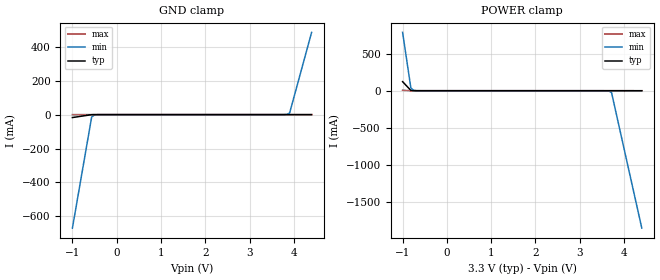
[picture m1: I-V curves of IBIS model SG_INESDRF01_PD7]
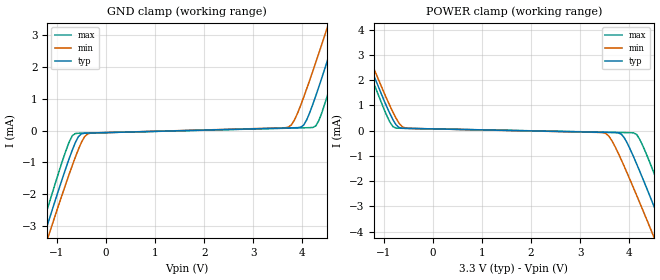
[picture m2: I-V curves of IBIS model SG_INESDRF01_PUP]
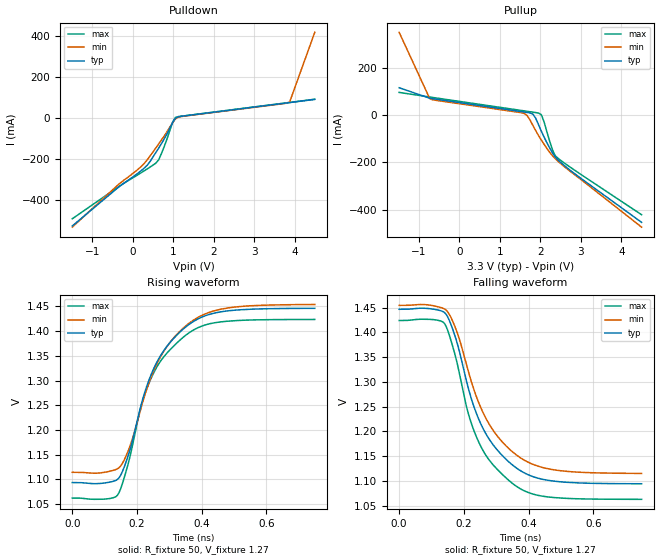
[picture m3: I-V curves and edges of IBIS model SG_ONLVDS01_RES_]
|   This file is an IBIS representation of the   |
|   Integrated Device Technology , Inc.   |
|   ICS854S058i   |
|   8:1 DIFFERENTIAL-TO-LVDS CLOCK MULTIPLIER   |
[IBIS Ver]   4.1
[File name]   854s058i_3v3.ibs
[File Rev]   1.0
[Date]   15 Jan 2010
[Source]   Originated at Integrated Device Technology, Inc.
[Disclaimer]
IDT hereby grants the user of this IBIS model a non-exclusive,
nontransferable license to use this IBIS model under the following terms.
Before using this IBIS model, the user should read this license.
If the user does not accept these terms,  the IBIS model should be
returned to IDT within 30 days.
   The user is granted this license only to use the IBIS model and
is not granted rights to sell, load, rent, lease or license the IBIS
model in whole or in part, or in modified form to anyone other than
user. User may modify the IBIS model to suit its specific
applications but rights to derivative works and such modifications
shall belong to IDT.
   This IBIS model is provided on an "AS IS" basis and IDT makes
absolutely no warranty with respect to the information contained
herein. IDT DISCLAIMS AND CUSTOMER WAIVES ALL WARRANTIES, EXPRESS
OR IMPLIED, INCLUDING WARRANTIES OF MERCHANTABILITY OR FITNESS FOR
A PARTICULAR PURPOSE. The entire risk as to quality and performance
is with the Customer. ACCORDINGLY, IN NO EVENT SHALL THE COMPANY BE
LIABLE FOR ANY DAMAGES, WHETHER IN CONTRACT OR TORT,INCLUDING ANY
LOST PROFITS OR OTHER INCIDENTAL, CONSEQUENTIAL, EXEMPLARY, OR
PUNITIVE DAMAGES ARISING OUT OF THE USE OR APPLICATION OF THE IBIS
model provided in this package. Further, IDT reserves the right to
make changes without notice to any product herein to improve
reliability, function, or design. IDT does not convey any license
under patent rights or any other intellectual property rights,
including those of third parties.
   IDT is not obligated to provide maintenance or support
for the licensed IBIS model.
[Copyright]   Copyright 2010 by Integrated Device Technology, Inc.
[Component]   ICS854S058GI
[Manufacturer] Integrated Device Technology, Inc.
[Package]
|TSSOP 24 Lead
|   typ   min   max
R_pkg   60.65m   52.4m   68.9m
L_pkg   1.989nH   1.431nH   2.547nH
C_pkg   0.314pF   0.254pF   0.374pF
[Pin] signal_name  model_name   R_pin   L_pin   C_pin
1   PCLK0   SG_INESDRF01_PD7   68.9m   2.547n   0.374p
2   nPCLKO   SG_INESDRF01_PUP   65.6m   2.323n   0.350p
3   PCLK1   SG_INESDRF01_PD7   62.3m   2.100n   0.326p
4   nPCLK1   SG_INESDRF01_PUP   59.0m   1.877n   0.302p
5   VDD   POWER   55.7m   1.654n   0.278p
6   SELO   SG_INESDRF01_PD7   52.4m   1.431n   0.254p
7   SEL1   SG_INESDRF01_PD7   52.4m   1.431n   0.254p
8   SEL2   SG_INESDRF01_PD7   55.7m   1.654n   0.278p
9   PCLK2   SG_INESDRF01_PD7   59.0m   1.877n   0.302p
10  nPCLK2   SG_INESDRF01_PUP   62.3m   2.100n   0.326p
11  PCLK3   SG_INESDRF01_PD7   65.6m   2.323n   0.350p
12  nPCLK3   SG_INESDRF01_PUP   68.9m   2.547n   0.374p
13  nPCLK4   SG_INESDRF01_PD7   68.9m   2.547n   0.374p
14  PCLK4   SG_INESDRF01_PUP   65.6m   2.323n   0.350p
15  nPCLK5   SG_INESDRF01_PD7   62.3m   2.100n   0.326p
16  PCLK5   SG_INESDRF01_PUP   59.0m   1.877n   0.302p
17  GND   GND   55.7m   1.654n   0.278p
18  nQ   SG_ONLVDS01_RES_   52.4m   1.431n   0.254p
19  Q   SG_ONLVDS01_RES_   52.4m   1.431n   0.254p
20  VDD   POWER   55.7m   1.654n   0.278p
21  nPCLK6   SG_INESDRF01_PD7   59.0m   1.877n   0.302p
22  PCLK6   SG_INESDRF01_PUP   62.3m   2.100n   0.326p
23  nPCLK7   SG_INESDRF01_PD7   65.6m   2.323n   0.350p
24  PCLK7   SG_INESDRF01_PUP   68.9m   2.547n   0.374p
[Diff Pin]  inv_pin  vdiff tdelay_typ tdelay_min  tdelay_max
1   2   NA   0   0   0
3   4   NA   0   0   0
9   10   NA   0   0   0
11   12   NA   0   0   0
14   13   NA   0   0   0
16   15   NA   0   0   0
22   21   NA   0   0   0
24   23   NA   0   0   0
19   18   0.15   0   0   0
| Models and submodels in the file (3): SG_INESDRF01_PD7 (Input), SG_INESDRF01_PUP (Input), SG_ONLVDS01_RES_ (Output)
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[Model]   SG_INESDRF01_PD7
Model_type   Input
Polarity   Non-Inverting
Vinl = 0.8V
Vinh = 2.0V
|   typ   min   max
C_comp   2pF   1.5pF   2.5pF
|   typ   min   max
[Voltage range]   3.3V   3.135V   3.465V
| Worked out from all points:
|   GND clamp passes 1 mA (typ) near -0.58 V on its own axis
|   POWER clamp passes 1 mA (typ) near -0.76 V on its own axis
[GND_clamp]
|Voltage   I (typ)   I (min)   I (max)
-999mV    -17.25mA   -669.4mA   -57.61uA
-564.6mV  -245.6uA   -14.47mA   -7.295uA
-502.5mV  -27.9uA    -1.943mA   -6.234uA
-378.4mV  -5.16uA    -39.86uA   -4.684uA
3.841V    50.75uA    1.283mA    47.55uA
3.904V    52.59uA    9.247mA    48.31uA
4.4V      150.7uA    485.1mA    54.46uA
[Power_clamp]
|Voltage   I (typ)   I (min)   I (max)
-999mV    122.4mA    788mA      6.109mA
-812.8mV  3.927mA    38.66mA    147.8uA
-750.8mV  399.4uA    5.222mA    56.5uA
3.593V    -3.873uA   -467.3uA   -1.587uA
3.655V    -4.754uA   -3.451mA   -2.355uA
3.717V    -6.276uA   -25.73mA   -3.124uA
4.4V      -102uA     -1.856A    -11.57uA
[Model]   SG_INESDRF01_PUP
Model_type   Input
Polarity   Non-Inverting
Vinl = 0.8V
Vinh = 2.0V
|   typ   min   max
C_comp   2pF   1.5pF   2.5pF
|   typ   min   max
[Voltage range]   3.3V   3.135V   3.465V
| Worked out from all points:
|   GND clamp passes 1 mA (typ) near -0.78 V on its own axis
|   POWER clamp passes 1 mA (typ) near -0.95 V on its own axis
[GND_clamp]
|Voltage   I (typ)   I (min)   I (max)
-3.3V     -13.37mA   -13.5mA    -13.23mA
-1.46V    -4.238mA   -4.649mA   -3.775mA
-1V       -2.017mA   -2.491mA   -1.48mA
-626.7mV  -377uA     -836uA     -94.14uA
-316.4mV  -78uA      -81.69uA   -76.26uA
3.717V    81.99uA    107.5uA    73.88uA
4.028V    171.5uA    1.045mA    85.43uA
4.214V    823.3uA    1.864mA    96.14uA
4.401V    1.668mA    2.722mA    570uA
4.841V    3.778mA    4.79mA     2.685mA
5.281V    5.937mA    6.89mA     4.912mA
6.6V      12.5mA     13.26mA    11.7mA
[Power_clamp]
|Voltage   I (typ)   I (min)   I (max)
-3.3V     12.5mA     12.46mA    12.55mA
-1.92V    5.638mA    5.81mA     5.445mA
-1.46V    3.385mA    3.629mA    3.108mA
-750.8mV  223.1uA    483.2uA    96.58uA
-502.5mV  85.39uA    86.45uA    83.19uA
3.469V    -72.15uA   -85.75uA   -64.64uA
3.841V    -147.4uA   -1.172mA   -78.5uA
4.09V     -1.046mA   -2.283mA   -93.51uA
4.401V    -2.497mA   -3.732mA   -1.172mA
4.841V    -4.634mA   -5.819mA   -3.349mA
5.281V    -6.803mA   -7.927mA   -5.587mA
6.6V      -13.37mA   -14.3mA    -12.38mA
[Model]   SG_ONLVDS01_RES_
Model_type   Output
Polarity   Non-Inverting
|   typ   min   max
C_comp   2pF   1.5pF   2.5pF
Vmeas = 1.27V
Rref = 50
Cref = 0
Vref = 1.27V
|   typ   min   max
[Voltage range]   3.3V   3.135V   3.465V
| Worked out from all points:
|   slope of the pulldown table from 0 to 0.495 V, typ, clamps not added: 5.18 ohm
|   slope of the pullup table from 0 to 0.495 V, typ, clamps not added: 40 ohm
|   rising waveform, R_fixture 50, V_fixture 1.27: 20-80 % time 120ps typ, 127ps min, 113ps max; typ from 1.09 V to 1.45 V
|   falling waveform, R_fixture 50, V_fixture 1.27: 20-80 % time 120ps typ, 127ps min, 113ps max; typ from 1.45 V to 1.09 V
[Pulldown]
|Voltage   I (typ)   I (min)   I (max)
-1.49V    -526mA     -531.8mA   -491mA
-388.4mV  -343.7mA   -330.7mA   -340.3mA
300.1mV   -241.8mA   -218.4mA   -255.7mA
437.8mV   -210.2mA   -183.2mA   -238.2mA
575.5mV   -167.6mA   -145.3mA   -219.5mA
644.4mV   -146.5mA   -126.1mA   -203.8mA
713.2mV   -124.6mA   -106.8mA   -172.7mA
988.6mV   -22.01mA   -22.42mA   -20.11mA
1.057V    -1.019mA   -4.243mA   3.11mA
1.126V    6.082mA    4.308mA    6.981mA
3.88V     75.42mA    78.38mA    76.3mA
4.5V      90.95mA    418mA      91.88mA
[Pullup]
|Voltage   I (typ)   I (min)   I (max)
-1.49V    116.4mA    351.2mA    96.67mA
-732.6mV  71.96mA    69.82mA    77.06mA
1.608V    13.33mA    7.135mA    18.21mA
1.677V    11.59mA    -2.441mA   16.48mA
1.815V    4.596mA    -43.54mA   13.02mA
1.953V    -39.73mA   -85.83mA   9.331mA
2.021V    -67.05mA   -105.1mA   2.575mA
2.09V     -92.61mA   -123.3mA   -28.02mA
2.297V    -159.1mA   -171.3mA   -146.1mA
2.366V    -176.6mA   -183.7mA   -171.9mA
2.848V    -247.8mA   -252.4mA   -233.1mA
4.5V      -453.8mA   -474.1mA   -421.6mA
[Ramp]
|   typ   min   max
dV/dt_r   0.283/0.193n   0.272/0.203n   0.291/0.185n
dV/dt_f   0.283/0.193n   0.272/0.203n   0.291/0.185n
R_load =   50.0000
[Rising Waveform]
R_fixture = 50
V_fixture = 1.27   |Vcc_typ
V_fixture_min = 1.284 |Vcc_min
V_fixture_max = 1.243 |Vcc_max
C_fixture = 0.0p
| Time   typ   min   max
0s        1.094V     1.114V     1.062V
102.1ps   1.093V     1.115V     1.06V
141.1ps   1.101V     1.122V     1.069V
177.9ps   1.159V     1.167V     1.145V
210.2ps   1.244V     1.239V     1.242V
240.2ps   1.306V     1.301V     1.3V
288.3ps   1.365V     1.365V     1.352V
354.4ps   1.41V      1.412V     1.393V
477.5ps   1.441V     1.446V     1.42V
749.2ps   1.446V     1.454V     1.423V
[Falling Waveform]
R_fixture = 50
V_fixture = 1.27   |Vcc_typ
V_fixture_min = 1.284 |Vcc_min
V_fixture_max = 1.243 |Vcc_max
C_fixture = 0.0p
| Time   typ   min   max
0s        1.447V     1.454V     1.424V
102.1ps   1.447V     1.454V     1.426V
141.1ps   1.439V     1.447V     1.417V
177.9ps   1.381V     1.402V     1.341V
210.2ps   1.296V     1.33V      1.244V
240.2ps   1.234V     1.267V     1.187V
288.3ps   1.175V     1.204V     1.134V
354.4ps   1.13V      1.156V     1.093V
477.5ps   1.099V     1.122V     1.066V
749.2ps   1.094V     1.115V     1.063V
